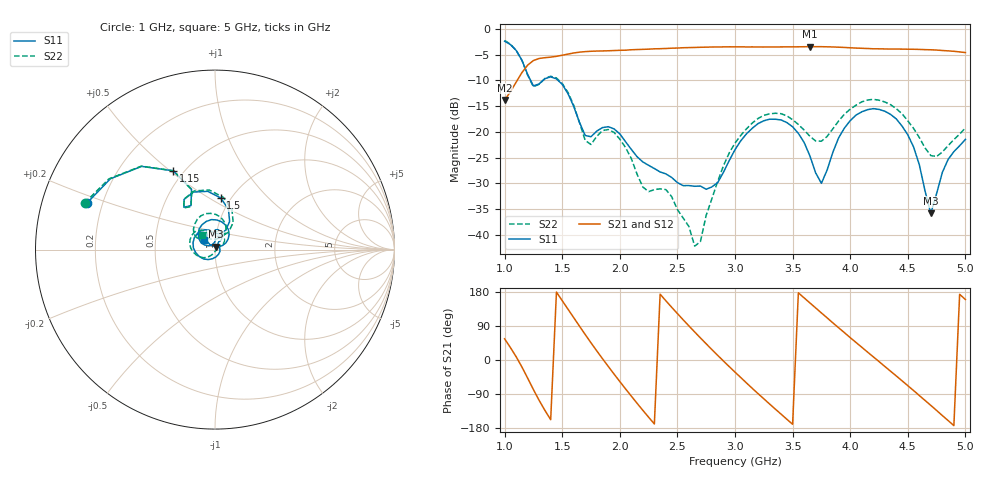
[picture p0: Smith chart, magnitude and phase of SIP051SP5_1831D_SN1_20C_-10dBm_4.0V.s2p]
# GHz  S  dB  R  50
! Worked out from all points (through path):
!   81 points, 1 GHz to 5 GHz, reference 50 ohm
!   highest |S21| = -3.46 dB at 3.65 GHz (marker M1); lowest = -13.8 dB at 1 GHz (marker M2)
!   lowest |S11| = -35.8 dB at 4.7 GHz (marker M3), VSWR 1.03, Z = 50.3 + j1.61 ohm
!   |S11| at or under -10 dB: 1.226 GHz to 1.333 GHz (107.7 MHz wide, 8.42 % of centre); 1.464 GHz to end of sweep
!   |S22| runs from -42.2 to -2.3 dB; largest |S21 - S12| = 0.0025
!   S11 on the Smith chart (normalised r, x): 1 GHz: 0.14, +0.17; 1.15 GHz: 0.44, +0.51; 1.5 GHz: 0.90, +0.56; 5 GHz: 0.88, +0.10
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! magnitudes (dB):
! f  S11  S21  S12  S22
! 1 GHz  -2.4  -13.8  -13.8  -2.3
! 1.15 GHz  -6.1  -8.5  -8.5  -6.1
! 1.25 GHz  -11.1  -6.1  -6.2  -11.2
! 1.5 GHz  -10.8  -5.1  -5.1  -10.6
! 1.7 GHz  -20.7  -4.4  -4.4  -21.7
! 1.95 GHz  -19.4  -4.2  -4.2  -20.1
! 2.2 GHz  -25.8  -4.0  -4.0  -30.7
! 2.35 GHz  -27.8  -3.9  -3.8  -31.0
! 2.65 GHz  -30.5  -3.6  -3.6  -42.2
! 2.7 GHz  -30.5  -3.6  -3.6  -41.3
! 2.85 GHz  -29.8  -3.5  -3.5  -29.6
! 3 GHz  -23.4  -3.5  -3.5  -22.2
! 3.35 GHz  -17.5  -3.5  -3.5  -16.4
! 3.65 GHz  -24.6  -3.5  -3.5  -20.8
! 3.7 GHz  -27.9  -3.5  -3.5  -21.8
! 3.75 GHz  -30.0  -3.5  -3.5  -21.8
! 4.05 GHz  -16.7  -3.7  -3.7  -14.8
! 4.35 GHz  -16.6  -3.9  -3.9  -14.7
! 4.55 GHz  -22.9  -4.0  -4.0  -19.3
! 4.7 GHz  -35.8  -4.1  -4.1  -24.6
! 4.85 GHz  -25.3  -4.3  -4.3  -22.7
! 5 GHz  -21.5  -4.6  -4.6  -19.2
